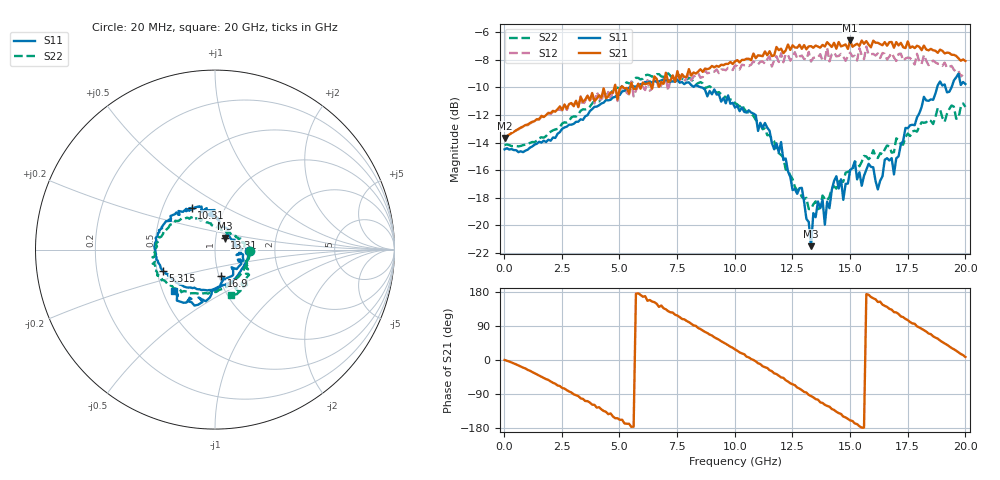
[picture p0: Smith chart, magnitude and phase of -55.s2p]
!Agilent Technologies,N5230A,US43500223,A.07.50.48
!Agilent N5230A: A.07.50.48
!Date: Wednesday, October 07, 2015 14:48:20
!Correction: S11(Full 2 Port(1,2))
!S21(Full 2 Port(1,2))
!S12(Full 2 Port(1,2))
!S22(Full 2 Port(1,2))
!S2P File: Measurements: S11, S21, S12, S22:
# Hz S  dB  R 50
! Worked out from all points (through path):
!   201 points, 20 MHz to 20 GHz, reference 50 ohm
!   highest |S21| = -6.60 dB at 15.01 GHz (marker M1); lowest = -13.7 dB at 20 MHz (marker M2)
!   group delay of S21, straight-line fit = 100 ps
!   lowest |S11| = -21.5 dB at 13.31 GHz (marker M3), VSWR 1.18, Z = 55.2 + j7.16 ohm
!   |S11| at or under -10 dB: start of sweep to 5.442 GHz; 8.549 GHz to 18.78 GHz (10.23 GHz wide, 74.9 % of centre); 19.14 GHz to 19.4 GHz (261.8 MHz wide, 1.36 % of centre)
!   |S22| runs from -18.8 to -9.0 dB; largest |S21 - S12| = 0.097
!   S11 on the Smith chart (normalised r, x): 20 MHz: 1.46, -0.02; 5.315 GHz: 0.54, -0.14; 10.31 GHz: 0.70, +0.35; 13.31 GHz: 1.10, +0.14; 16.9 GHz: 1.03, -0.31; 20 GHz: 0.57, -0.30
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2e7  -14.49 -1.5  -13.68 0.0  -13.69 -0.3  -14.18 -1.5
1.9181e9  -13.80 -73.7  -11.86 -52.7  -11.83 -54.2  -13.33 -70.4
3.4166e9  -12.35 -118.3  -11.04 -102.7  -11.31 -107.0  -11.59 -108.8
5.3147e9  -10.08 -157.2  -10.04 -168.3  -10.38 -169.2  -9.63 -143.5
6.7133e9  -9.57 -179.7  -9.97 140.1  -10.10 137.1  -9.04 -160.9
8.5115e9  -9.98 152.3  -8.68 81.8  -9.30 76.6  -9.61 174.3
1.001e10  -11.47 126.9  -8.11 28.0  -8.41 22.6  -11.14 149.3
1.03097e10  -11.46 119.0  -8.01 17.3  -8.35 12.7  -11.25 144.1
1.18082e10  -14.05 101.1  -7.07 -37.0  -7.74 -45.3  -14.49 116.5
1.29071e10  -17.28 55.3  -7.20 -79.6  -7.69 -88.0  -17.93 87.5
1.33067e10  -21.52 50.0  -7.01 -95.1  -8.13 -102.0  -18.82 72.5
1.34066e10  -19.12 45.9  -7.12 -98.7  -7.85 -104.9  -18.47 69.7
1.39061e10  -19.96 11.5  -7.04 -118.3  -7.94 -122.4  -18.09 46.6
1.43057e10  -16.78 2.7  -6.76 -131.8  -7.46 -137.2  -17.17 33.3
1.47053e10  -18.16 -14.2  -6.96 -149.3  -7.76 -156.0  -16.85 23.5
1.5005e10  -15.98 -10.0  -6.60 -159.5  -7.48 -163.3  -16.02 13.9
1.62038e10  -17.40 -46.7  -6.76 153.1  -7.54 147.7  -15.12 -6.9
1.67033e10  -15.30 -67.2  -6.72 135.0  -7.74 130.9  -14.28 -17.2
1.69031e10  -16.31 -76.6  -7.12 126.3  -7.82 116.7  -14.70 -20.9
1.82018e10  -10.68 -100.1  -6.97 78.8  -7.65 72.8  -12.57 -40.9
1.91009e10  -9.79 -117.4  -7.54 43.7  -8.20 34.5  -12.50 -50.6
2e10  -9.76 -134.7  -8.08 7.9  -9.03 -3.1  -11.41 -70.2
